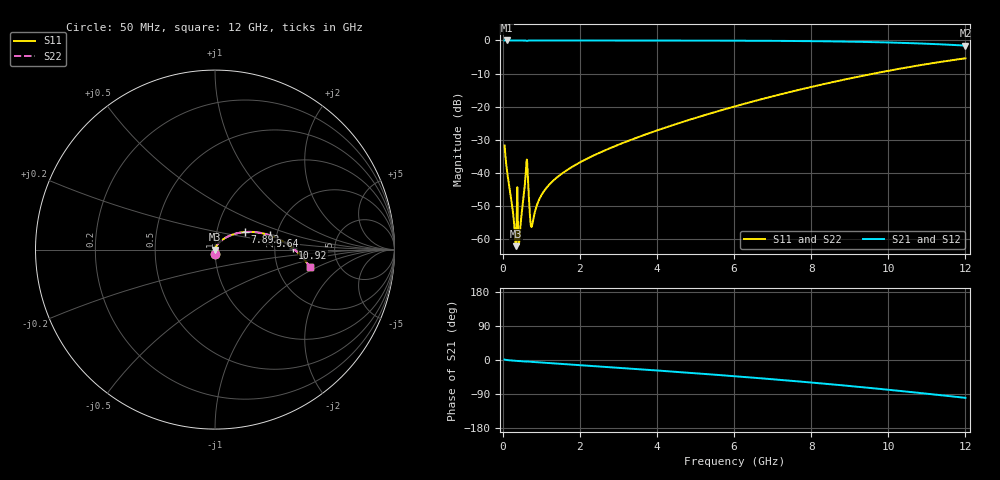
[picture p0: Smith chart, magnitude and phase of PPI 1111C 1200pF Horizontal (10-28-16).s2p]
# MHz S MA R 50
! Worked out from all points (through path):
!   1601 points, 50 MHz to 12 GHz, reference 50 ohm
!   highest |S21| = 0.00 dB at 102.3 MHz (marker M1); lowest = -1.5 dB at 12 GHz (marker M2)
!   group delay of S21, straight-line fit = 22.7 ps
!   lowest |S11| = -62.0 dB at 341.3 MHz (marker M3), VSWR 1.00, Z = 50.1 - j0.018 ohm
!   |S11| at or under -10 dB: start of sweep to 9.621 GHz
!   |S22| runs from -62.0 to -5.4 dB; largest |S21 - S12| = 0
!   S11 on the Smith chart (normalised r, x): 50 MHz: 1.00, -0.05; 7.892 GHz: 1.36, +0.28; 9.64 GHz: 1.85, +0.33; 10.92 GHz: 2.53, +0.06; 12 GHz: 3.07, -0.85
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50  0.02601 -88.1  0.9993 1.2  0.9993 1.2  0.02601 -88.1
102.2812  0.01206 -88.1  0.9995 0.0  0.9995 0.0  0.01206 -88.1
296.4688  0.001731 -70.2  0.9993 -1.8  0.9993 -1.8  0.001731 -70.2
341.2812  0.0007903 -13.1  0.9992 -2.2  0.9992 -2.2  0.0007903 -13.1
378.625  0.006117 -14.6  0.994 -2.3  0.994 -2.3  0.006117 -14.6
460.7812  0.001599 54.7  0.9991 -3.0  0.9991 -3.0  0.001599 54.7
572.8125  0.006481 65.3  0.9977 -4.0  0.9977 -4.0  0.006481 65.3
610.1562  0.01286 42.9  0.9912 -4.4  0.9912 -4.4  0.01286 42.9
654.9688  0.008392 -39.8  0.9932 -3.9  0.9932 -3.9  0.008392 -39.8
722.1875  0.00179 -17.5  0.9982 -4.6  0.9982 -4.6  0.00179 -17.5
767  0.001666 30.9  0.9986 -5.0  0.9986 -5.0  0.001666 30.9
938.7812  0.003904 67.3  0.9988 -6.2  0.9988 -6.2  0.003904 67.3
1147.906  0.006108 71.6  0.9988 -7.7  0.9988 -7.7  0.006108 71.6
2044.156  0.01491 70.7  0.9984 -13.9  0.9984 -13.9  0.01491 70.7
4038.312  0.04469 59.5  0.9968 -27.9  0.9968 -27.9  0.04469 59.5
6025  0.1015 45.6  0.9918 -42.9  0.9918 -42.9  0.1015 45.6
7892.188  0.1923 30.5  0.9774 -58.4  0.9774 -58.4  0.1923 30.5
8019.156  0.2001 29.4  0.9758 -59.6  0.9758 -59.6  0.2001 29.4
9639.875  0.3178 14.4  0.9433 -74.8  0.9433 -74.8  0.3178 14.4
10013.31  0.3496 10.6  0.9318 -78.6  0.9318 -78.6  0.3496 10.6
10924.5  0.433 1.2  0.8957 -88.1  0.8957 -88.1  0.433 1.2
12000  0.5379 -10.5  0.8366 -99.9  0.8366 -99.9  0.5379 -10.5
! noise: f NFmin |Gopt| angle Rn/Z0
50  0.0003799  0.8686  0.3351  0.0006219
1372  0.003962  0.6892  8.731  0.002465
2701  0.006448  0.6402  17.01  0.003314
4031  0.008736  0.6183  25.02  0.004075
5360  0.01097  0.6104  32.66  0.004832
6682  0.01323  0.6124  39.85  0.005641
8012  0.01561  0.6219  46.63  0.006568
9341  0.01819  0.6374  52.99  0.00767
1.067e+04  0.02105  0.6578  58.94  0.009023
1.2e+04  0.0243  0.6821  64.53  0.01073
